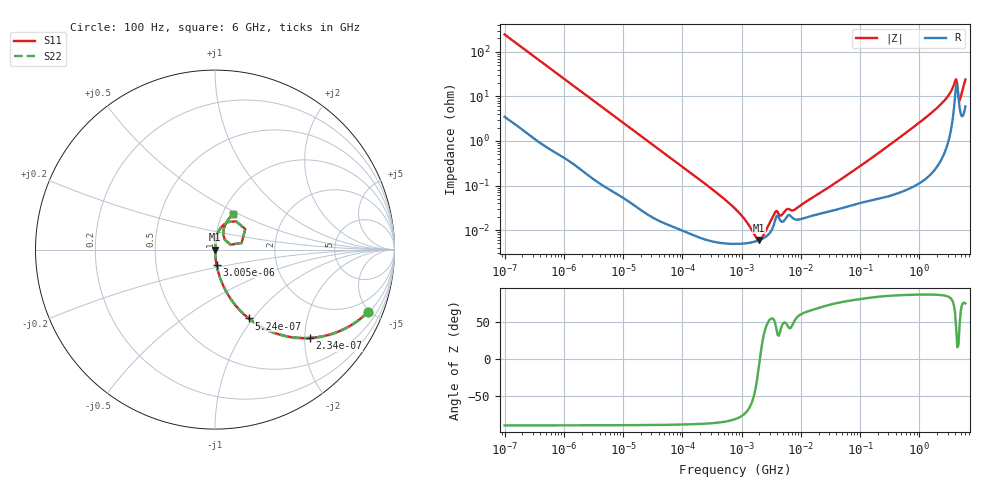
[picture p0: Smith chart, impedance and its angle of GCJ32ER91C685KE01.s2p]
!Murata Part Number: GCJ32ER91C685KE01
!These Parameters are Measured in Series Mode Connection
!Data Generated on Mar 13, 2026
!  o--ll--o
!Port1  Port2
!  o------o
!Operation Temp=25[degC], DC Bias Voltage=0[V]
!Freq. Start=100[Hz] Stop=6[GHz] 401[Steps]
# Hz S RI R 50
!Freq.(Hz) S11(Real) S11(Imag) S21(Real) S21(Imag) S12(Real) S12(Imag) S22(Real) S22(Imag)
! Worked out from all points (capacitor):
!   401 points, 100 Hz to 6 GHz, reference 50 ohm
!   read as one part in series: C = 6.46 uF near 109 Hz
!   lowest |Z| = 5.96 mohm at 1.983 MHz (marker M1)
!   series resonance near 2.034 MHz, so ESL is about 950 pH
!   S11 on the Smith chart (normalised r, x): 100 Hz: 1.07, -4.91; 234 Hz: 1.03, -2.11; 524 Hz: 1.01, -0.95; 3.005 kHz: 1.00, -0.17; 6 GHz: 1.12, +0.46
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100  0.8543 -0.3458  0.1457 0.3458  0.1457 0.3458  0.8543 -0.3458
234  0.5275 -0.4921  0.4725 0.4921  0.4725 0.4921  0.5275 -0.4921
524  0.1879 -0.3833  0.8121 0.3833  0.8121 0.3833  0.1879 -0.3833
2008  0.0177 -0.1234  0.9823 0.1234  0.9823 0.1234  0.0177 -0.1234
3005  0.00851 -0.0837  0.9915 0.0837  0.9915 0.0837  0.00851 -0.0837
40335  0.000203 -0.00648  0.9998 0.00648  0.9998 0.00648  0.000203 -0.00648
774597  4.89e-05 -0.000299  1 0.000299  1 0.000299  4.89e-05 -0.000299
1449809  5.26e-05 -9.29e-05  0.9999 9.29e-05  0.9999 9.29e-05  5.26e-05 -9.29e-05
1983483  5.92e-05 -6.8e-06  0.9999 6.8e-06  0.9999 6.8e-06  5.92e-05 -6.8e-06
2594782  7.18e-05 6.99e-05  0.9999 -6.99e-05  0.9999 -6.99e-05  7.18e-05 6.99e-05
3712478  0.00017 0.00019  0.9998 -0.00019  0.9998 -0.00019  0.00017 0.00019
4643984  0.000156 0.000142  0.9998 -0.000142  0.9998 -0.000142  0.000156 0.000142
5809218  0.000199 0.000215  0.9998 -0.000215  0.9998 -0.000215  0.000199 0.000215
7599586  0.000179 0.000215  0.9998 -0.000215  0.9998 -0.000215  0.000179 0.000215
1.555665e7  0.000209 0.000488  0.9998 -0.000488  0.9998 -0.000488  0.000209 0.000488
3.124326e8  0.000644 0.00805  0.9994 -0.00805  0.9994 -0.00805  0.000644 0.00805
1.95892e9  0.00542 0.0535  0.9946 -0.0535  0.9946 -0.0535  0.00542 0.0535
2.931063e9  0.0162 0.092  0.9838 -0.092  0.9838 -0.092  0.0162 0.092
3.8344e9  0.075 0.1541  0.925 -0.1541  0.925 -0.1541  0.075 0.1541
4.009986e9  0.1173 0.1571  0.8827 -0.1571  0.8827 -0.1571  0.1173 0.1571
5.016141e9  0.0459 0.0826  0.9541 -0.0826  0.9541 -0.0826  0.0459 0.0826
6e9  0.0991 0.1968  0.9009 -0.1968  0.9009 -0.1968  0.0991 0.1968
